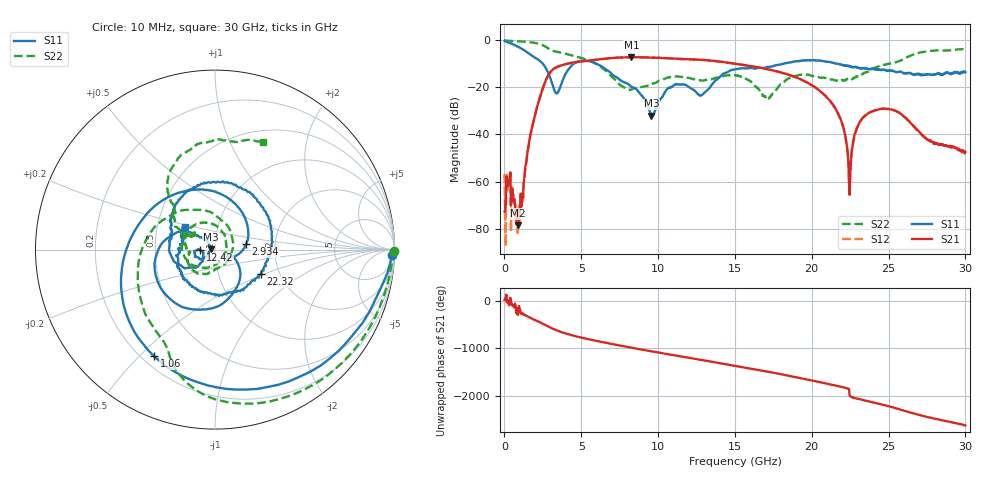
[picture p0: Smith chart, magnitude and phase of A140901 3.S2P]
!  2-Port S-parameters saved by WinCal
! VAR MeasName=S-Parameters (CALIBRATED_DATA) read from VNA (N5244A)
! VAR MeasDate=11/3/2014 9:26:44 AM
! VAR NAME=A140901 3
! VAR FILENAME=A140901 3.S2P
! VAR DATE=11/3/2014 9:26:44 AM
! VAR PHYS_PORTS=1,2
# Hz S RI R 50
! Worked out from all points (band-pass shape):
!   801 points, 10 MHz to 30 GHz, reference 50 ohm
!   highest |S21| = -7.11 dB at 8.257 GHz (marker M1); lowest = -78.5 dB at 872.2 MHz (marker M2)
!   |S21| within 3 dB of the highest: 3.966 GHz to 15.2 GHz (11.23 GHz wide, 117 % of centre)
!   lowest |S11| = -32.1 dB at 9.569 GHz (marker M3), VSWR 1.05, Z = 47.6 + j0.26 ohm
!   |S11| at or under -10 dB: 2.511 GHz to 4.496 GHz (1.986 GHz wide, 56.7 % of centre); 6.019 GHz to 18.13 GHz (12.11 GHz wide, 100 % of centre); 21.74 GHz to end of sweep
!   |S22| runs from -24.7 to 0.0 dB; largest |S21 - S12| = 0.0038
!   S11 on the Smith chart (normalised r, x): 10 MHz: 21, -54; 1.06 GHz: 0.25, -0.55; 2.934 GHz: 1.42, +0.09; 12.42 GHz: 0.85, -0.00; 22.32 GHz: 1.61, -0.48; 30 GHz: 0.69, +0.18
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1e7  0.9869 -0.0318  0.000217 7.3e-05  -0.000753 -0.00121  0.998 -0.00838
2.724125e8  0.7386 -0.5117  0.000433 -0.000959  0.000939 -0.000648  0.9645 -0.1776
8.722125e8  -0.1368 -0.7245  5.35e-05 0.000105  -5.51e-05 5.96e-05  0.8119 -0.5102
1.05965e9  -0.3394 -0.5948  -8.75e-05 0.000544  -9.08e-05 0.00047  0.7395 -0.5984
1.771912e9  -0.4748 0.052  0.0128 -0.003  0.0128 -0.003  0.3631 -0.8316
2.934025e9  0.1733 0.0298  -0.1937 0.0501  -0.1934 0.0497  -0.2506 -0.6004
3.421362e9  0.068 -0.0313  -0.0175 0.2711  -0.0181 0.2707  -0.3107 -0.4787
5.033325e9  -0.2176 -0.3004  0.187 -0.306  0.1869 -0.3063  -0.4197 -0.0391
6.75775e9  -0.2031 0.0993  -0.4147 -0.0333  -0.4144 -0.0339  -0.0168 0.2051
8.25725e9  -0.0782 0.0678  -0.00998 0.4408  -0.0099 0.4394  0.0739 -0.051
9.569312e9  -0.0248 0.00273  0.4182 0.1065  0.4171 0.1064  -0.00786 -0.1182
1.001916e10  -0.0391 -0.0306  0.4192 -0.0824  0.4183 -0.0824  -0.0371 -0.1319
1.241836e10  -0.0836 -0.00273  -0.3188 -0.2288  -0.3187 -0.2279  -0.1458 -0.0248
1.5005e10  -0.2373 -0.0484  0.114 0.2979  0.1161 0.2967  -0.1327 0.1229
1.714179e10  -0.2463 0.1181  0.1408 -0.1999  0.1397 -0.1992  0.0545 -0.0271
2.002832e10  0.0693 0.3755  -0.0531 0.0963  -0.0538 0.096  -0.1591 0.073
2.171526e10  0.3161 0.0176  0.028 -0.000329  0.0277 -6.57e-05  -0.1121 0.0882
2.231506e10  0.2572 -0.1361  0.00328 -0.00364  0.00336 -0.00358  -0.1239 0.081
2.25025e10  0.2212 -0.166  -0.00112 0.000715  -0.00123 0.000768  -0.1324 0.0698
2.336471e10  0.0406 -0.2543  0.0102 0.021  0.0102 0.0212  -0.1775 0.0905
2.501416e10  -0.1939 -0.1104  0.0148 -0.0314  0.0149 -0.0316  -0.2266 0.2261
3e10  -0.1691 0.1265  -0.00148 -0.00395  -0.00108 -0.00381  0.2701 0.6021
